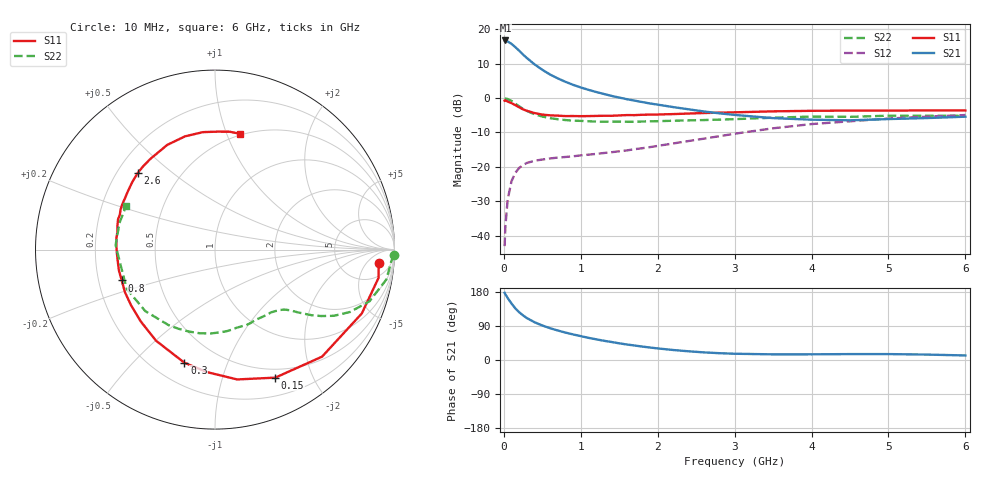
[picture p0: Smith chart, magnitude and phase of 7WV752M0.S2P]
! Infineon Technologies  Discrete & RF Semiconductors
! BFS17W
! Si NPN RF Bipolar Junction Transistor in SOT323
! VCE = 0.75 V  IC = 2 mA
! Common Emitter S-Parameters:  August  1999
# GHz  S  MA  R  50
!  f  S11  S21  S12  S22
! GHz  MAG  ANG  MAG  ANG  MAG  ANG  MAG  ANG
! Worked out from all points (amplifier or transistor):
!   36 points, 10 MHz to 6 GHz, reference 50 ohm
!   highest |S21| = 16.8 dB at 20 MHz (marker M1)
!   |S21| within 3 dB of that: start of sweep to 199.6 MHz
!   unconditionally stable (mu >= 1): 740.1 MHz to end of sweep
!   at 250 MHz: K = 0.39, MSG = 16.1 dB, |S12| = -19.5 dB
!   at 1.4 GHz: K = 1.42, MAG = 4.3 dB, |S12| = -15.8 dB
!   at 6 GHz: K = 1.14, MAG = -2.5 dB, |S12| = -4.9 dB
!   S11 on the Smith chart (normalised r, x): 10 MHz: 12, -11; 150 MHz: 0.40, -1.50; 300 MHz: 0.32, -0.71; 800 MHz: 0.30, -0.15; 2.6 GHz: 0.28, +0.38; 6 GHz: 0.49, +1.12
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0.01  0.9152 -4.7  6.849 177.4  0.007 88.2  0.9962 -1.6
0.02  0.9247 -9.8  6.895 173.4  0.0134 85.0  0.9836 -4.0
0.05  0.892 -23.5  6.674 163.5  0.0335 77.1  0.9693 -9.9
0.1  0.8436 -45.0  6.144 149.0  0.0619 65.1  0.9077 -18.5
0.15  0.7884 -64.8  5.511 136.0  0.082 55.3  0.8288 -24.8
0.2  0.7339 -80.3  4.877 125.9  0.0964 49.2  0.7585 -29.1
0.25  0.6843 -93.6  4.297 117.6  0.1062 43.5  0.6966 -32.1
0.3  0.653 -105.1  3.824 110.6  0.1139 40.2  0.6504 -34.2
0.4  0.6047 -122.9  3.091 99.5  0.1226 35.3  0.5801 -37.1
0.5  0.5754 -136.1  2.58 91.1  0.1276 33.1  0.5392 -38.9
0.6  0.5611 -146.5  2.206 84.0  0.1322 32.3  0.511 -40.8
0.8  0.5473 -161.7  1.727 72.4  0.1389 32.5  0.479 -45.8
1.1  0.547 -178.1  1.319 58.5  0.1502 35.3  0.4595 -54.1
1.3  0.553 173.2  1.148 50.8  0.1587 38.0  0.4522 -61.0
1.6  0.5657 162.7  0.963 40.9  0.1732 41.6  0.452 -71.2
2.2  0.5849 145.7  0.74 26.4  0.2185 47.7  0.4681 -92.9
2.6  0.6062 135.3  0.639 20.1  0.2568 49.2  0.4791 -107.5
3.5  0.6412 114.5  0.511 14.9  0.3634 45.7  0.518 -138.6
4  0.6527 104.8  0.485 15.0  0.4187 40.5  0.5384 -156.0
4.5  0.6579 95.9  0.475 15.6  0.4591 35.1  0.533 -170.9
5.5  0.6619 82.9  0.512 14.3  0.5357 24.7  0.5525 164.4
6  0.6597 77.8  0.536 12.0  0.5665 19.6  0.5519 153.6
